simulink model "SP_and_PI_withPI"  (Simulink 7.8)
settings: Solver=ode15s  StartTime=0.0  StopTime=50  RelTol=1e-6
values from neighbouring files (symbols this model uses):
  delay = delayv(i)    [example.m]    (also in IAE_Simulink.m; Robustness_SP.m; Robustness_SP_P.m; Robustness_SP_PI.m)
libraries: simulink x2

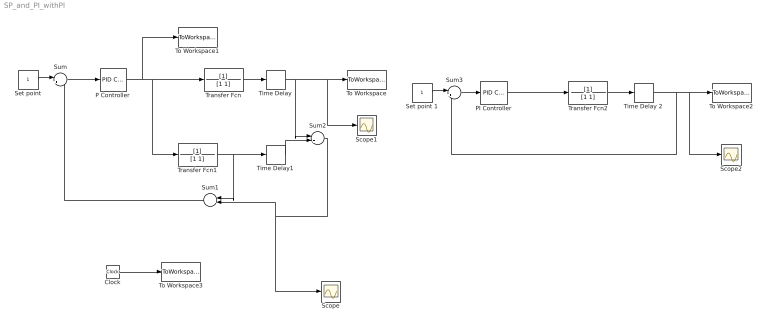
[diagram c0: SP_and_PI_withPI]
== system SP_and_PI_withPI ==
  Clock : Clock
  P Controller : simulink/Continuous/PID Controller  Controller=PI  TimeDomain=Continuous-time  SampleTime=1  IntegratorMethod=Forward Euler  FilterMethod=Forward Euler  Form=Ideal  P=2  I=1  D=0  N=100  InitialConditionSource=internal  InitialConditionForIntegrator=0  InitialConditionForFilter=0  ExternalReset=none  LimitOutput=off  UpperSaturationLimit=inf  LowerSaturationLimit=-inf  LinearizeAsGain=off  AntiWindupMode=none  Kb=1  TrackingMode=off  Kt=1  PParamMin=[]  PParamMax=[]  IParamMin=[]  IParamMax=[]  DParamMin=[]  DParamMax=[]  NParamMin=[]  NParamMax=[]  KbParamMin=[]  KbParamMax=[]  KtParamMin=[]  KtParamMax=[]  POutMin=[]  POutMax=[]  IOutMin=[]  IOutMax=[]  DOutMin=[]  DOutMax=[]  NOutMin=[]  NOutMax=[]  KbOutMin=[]  KbOutMax=[]  KtOutMin=[]  KtOutMax=[]  IntegratorOutMin=[]  IntegratorOutMax=[]  FilterOutMin=[]  FilterOutMax=[]  SumOutMin=[]  SumOutMax=[]  SumI1OutMin=[]  SumI1OutMax=[]  SumI2OutMin=[]  SumI2OutMax=[]  SumI3OutMin=[]  SumI3OutMax=[]  SumDOutMin=[]  SumDOutMax=[]  SaturationOutMin=[]  SaturationOutMax=[]  IntegratorContinuousStateAttributes=''  IntegratorStateMustResolveToSignalObject=off  IntegratorRTWStateStorageClass=Auto  FilterContinuousStateAttributes=''  FilterStateMustResolveToSignalObject=off  FilterRTWStateStorageClass=Auto
  PI Controller : simulink/Continuous/PID Controller  Controller=PI  TimeDomain=Continuous-time  SampleTime=1  IntegratorMethod=Forward Euler  FilterMethod=Forward Euler  Form=Ideal  P=0.5  I=1  D=0  N=100  InitialConditionSource=internal  InitialConditionForIntegrator=0  InitialConditionForFilter=0  ExternalReset=none  LimitOutput=off  UpperSaturationLimit=inf  LowerSaturationLimit=-inf  LinearizeAsGain=off  AntiWindupMode=none  Kb=1  TrackingMode=off  Kt=1  PParamMin=[]  PParamMax=[]  IParamMin=[]  IParamMax=[]  DParamMin=[]  DParamMax=[]  NParamMin=[]  NParamMax=[]  KbParamMin=[]  KbParamMax=[]  KtParamMin=[]  KtParamMax=[]  POutMin=[]  POutMax=[]  IOutMin=[]  IOutMax=[]  DOutMin=[]  DOutMax=[]  NOutMin=[]  NOutMax=[]  KbOutMin=[]  KbOutMax=[]  KtOutMin=[]  KtOutMax=[]  IntegratorOutMin=[]  IntegratorOutMax=[]  FilterOutMin=[]  FilterOutMax=[]  SumOutMin=[]  SumOutMax=[]  SumI1OutMin=[]  SumI1OutMax=[]  SumI2OutMin=[]  SumI2OutMax=[]  SumI3OutMin=[]  SumI3OutMax=[]  SumDOutMin=[]  SumDOutMax=[]  SaturationOutMin=[]  SaturationOutMax=[]  IntegratorContinuousStateAttributes=''  IntegratorStateMustResolveToSignalObject=off  IntegratorRTWStateStorageClass=Auto  FilterContinuousStateAttributes=''  FilterStateMustResolveToSignalObject=off  FilterRTWStateStorageClass=Auto
  Scope : Scope
  Scope1 : Scope
  Scope2 : Scope
  Set point : Constant
  Set point 1 : Constant
  Sum : Sum  Inputs=|+-
  Sum1 : Sum  Inputs=|++
  Sum2 : Sum  Inputs=|+-
  Sum3 : Sum  Inputs=|+-
  Time Delay 2 : TransportDelay  DelayTime=delay
  Time Delay1 : TransportDelay
  Time Delay : TransportDelay  DelayTime=delay
  To Workspace : ToWorkspace  VariableName=Ysp  SampleTime=-1  SaveFormat=Array
  To Workspace1 : ToWorkspace  VariableName=usp  SampleTime=-1  SaveFormat=Structure
  To Workspace2 : ToWorkspace  VariableName=Ypi  SampleTime=-1  SaveFormat=Array
  To Workspace3 : ToWorkspace  VariableName=time  SampleTime=-1  SaveFormat=Array
  Transfer Fcn : TransferFcn  Denominator=[1 1]
  Transfer Fcn1 : TransferFcn  Denominator=[1 1]
  Transfer Fcn2 : TransferFcn  Denominator=[1 1]
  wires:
  Set point/1 -> Sum/1
  Sum/1 -> P Controller/1
  P Controller/1 -> Transfer Fcn/1, Transfer Fcn1/1, To Workspace1/1
  Transfer Fcn/1 -> Time Delay/1
  Transfer Fcn1/1 -> Time Delay1/1, Sum1/1
  Time Delay/1 -> Sum2/1, To Workspace/1, Scope1/1
  Time Delay1/1 -> Sum2/2
  Sum2/1 -> Sum1/2, Scope/1
  Sum1/1 -> Sum/2
  Transfer Fcn2/1 -> Time Delay 2/1
  PI Controller/1 -> Transfer Fcn2/1
  Sum3/1 -> PI Controller/1
  Set point 1/1 -> Sum3/1
  Time Delay 2/1 -> Sum3/2, To Workspace2/1, Scope2/1
  Clock/1 -> To Workspace3/1
